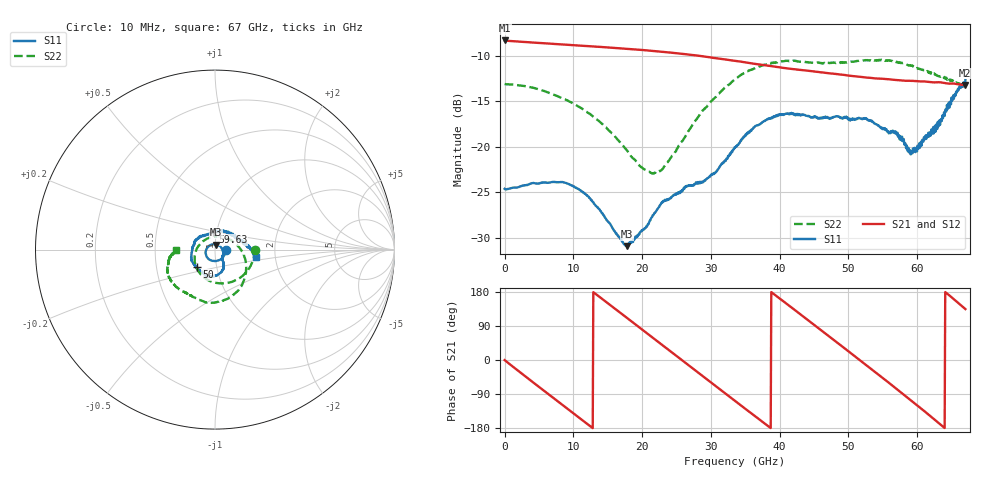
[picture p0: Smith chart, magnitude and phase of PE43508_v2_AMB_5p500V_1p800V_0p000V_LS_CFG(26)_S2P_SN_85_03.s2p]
!Keysight Technologies,N5227A,US51270237,A.10.43.00
!Date: Wednesday, August 22, 2018 17:09:15
!Correction: S11(Full 2 Port(1,3))
!S31(Full 2 Port(1,3))
!S13(Full 2 Port(1,3))
!S33(Full 2 Port(1,3))
!S2P File: Measurements: S11, S31, S13, S33:
# Hz S  dB  R 50
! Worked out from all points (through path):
!   801 points, 10 MHz to 67 GHz, reference 50 ohm
!   highest |S21| = -8.29 dB at 10 MHz (marker M1); lowest = -13.2 dB at 66.92 GHz (marker M2)
!   group delay of S21, straight-line fit = 38.9 ps
!   lowest |S11| = -30.9 dB at 17.76 GHz (marker M3), VSWR 1.06, Z = 50.2 + j2.85 ohm
!   |S11| at or under -10 dB: start of sweep to end of sweep
!   |S22| runs from -22.9 to -10.4 dB; largest |S21 - S12| = 0.0022
!   S11 on the Smith chart (normalised r, x): 10 MHz: 1.13, -0.00; 50 GHz: 0.80, -0.16; 59.63 GHz: 0.96, +0.19; 67 GHz: 1.59, -0.14
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1e7  -24.60 -0.7  -8.29 -0.2  -8.29 -0.2  -13.07 -0.3
2.522125e9  -24.29 -40.0  -8.44 -36.2  -8.43 -36.1  -13.26 -27.8
5.787888e9  -23.92 -85.7  -8.60 -81.9  -8.60 -81.9  -13.86 -62.0
8.300012e9  -23.87 -118.7  -8.72 -116.9  -8.72 -116.9  -14.62 -87.5
1.123082e10  -24.89 -154.8  -8.87 -157.7  -8.86 -157.6  -15.76 -116.2
1.424538e10  -27.30 162.1  -9.02 160.5  -9.01 160.5  -17.50 -147.0
1.776235e10  -30.91 84.0  -9.20 111.6  -9.20 111.6  -20.33 170.0
2.002326e10  -29.20 29.5  -9.34 80.0  -9.34 80.1  -22.30 132.0
2.236791e10  -26.69 -12.1  -9.50 47.4  -9.50 47.4  -22.69 84.3
2.47963e10  -25.25 -35.8  -9.68 13.4  -9.68 13.5  -20.56 40.0
2.714095e10  -24.20 -49.0  -9.88 -19.3  -9.88 -19.2  -17.80 9.1
3.040671e10  -23.00 -53.4  -10.21 -64.9  -10.19 -64.8  -14.71 -21.4
3.3505e10  -20.08 -61.0  -10.53 -107.9  -10.53 -107.9  -12.57 -46.8
3.88642e10  -16.85 -89.0  -11.12 178.0  -11.13 178.1  -10.79 -82.7
4.472582e10  -16.73 -118.6  -11.67 96.8  -11.65 96.8  -10.74 -111.6
5.000129e10  -17.01 -136.9  -12.14 22.9  -12.15 22.8  -10.65 -127.4
5.284836e10  -17.00 -157.5  -12.38 -17.2  -12.38 -17.3  -10.49 -137.1
5.586291e10  -18.51 166.6  -12.56 -60.0  -12.57 -60.2  -10.49 -149.3
5.96311e10  -20.09 97.7  -12.75 -114.2  -12.78 -114.4  -11.27 -162.3
6.339929e10  -17.00 29.6  -12.90 -170.4  -12.95 -170.7  -12.28 -173.1
6.691626e10  -13.11 -8.7  -13.19 135.8  -13.25 135.9  -13.11 -178.1
6.7e10  -12.65 -10.1  -13.18 134.4  -13.24 134.5  -13.19 -179.1
